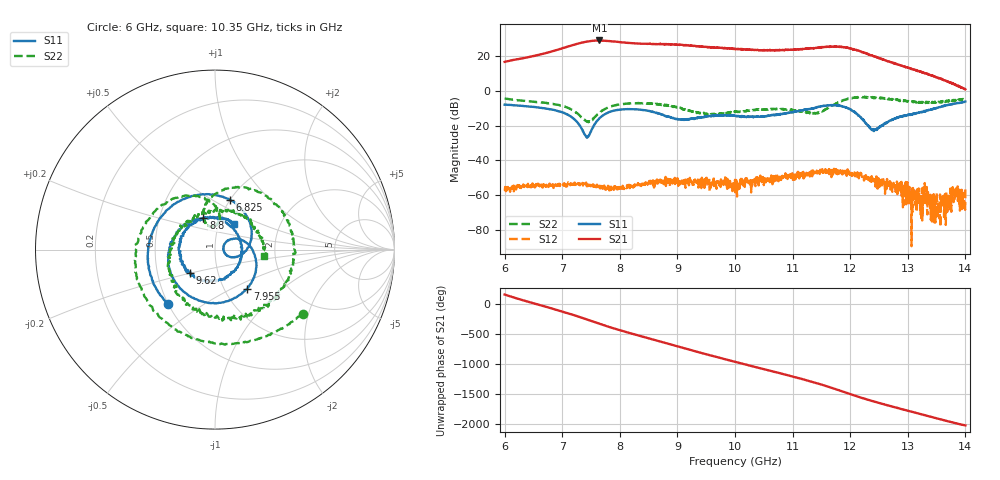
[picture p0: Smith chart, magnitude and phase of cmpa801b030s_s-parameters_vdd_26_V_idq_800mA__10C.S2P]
!Keysight Technologies,E5071C,MY46110325,B.14.03
!Date: Fri Aug 07 13:49:55 2020
!Data & Calibration Information:
!Freq	S11:SOLT2(ON)	S21:SOLT2(ON)	S12:SOLT2(ON)	S22:SOLT2(ON)
!PortZ  Port1:50+j0  Port2:50+j0
!Above PortZ is port z conversion or system Z0 setting when saving the data.
!When reading, reference impedance value at option line is always used.
# Hz S dB R 50
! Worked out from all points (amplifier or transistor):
!   1601 points, 6 GHz to 14 GHz, reference 50 ohm
!   highest |S21| = 29.0 dB at 7.645 GHz (marker M1)
!   |S21| within 3 dB of that: 7.15 GHz to 9.222 GHz (2.072 GHz wide, 25.3 % of centre)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
!   unconditionally stable (mu >= 1): start of sweep to end of sweep
!   at 7.33 GHz: K = 9.77, MAG = 27.8 dB, |S12| = -53.7 dB
!   at 10 GHz: K = 10.16, MAG = 24.5 dB, |S12| = -51.1 dB
!   at 14 GHz: K = 123.78, MAG = 4.0 dB, |S12| = -55.0 dB
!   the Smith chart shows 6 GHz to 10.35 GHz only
!   S11 on the Smith chart (normalised r, x): 6 GHz: 0.50, -0.36; 6.825 GHz: 1.00, +0.60; 7.955 GHz: 1.27, -0.61; 8.8 GHz: 0.83, +0.30; 9.62 GHz: 0.74, -0.20; 10.35 GHz: 1.19, +0.35
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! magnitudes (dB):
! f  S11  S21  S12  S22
! 6 GHz  -7.9  16.6  -57.3  -4.3
! 6.825 GHz  -10.8  22.7  -54.0  -7.5
! 7.335 GHz  -21.6  27.7  -54.0  -15.1
! 7.445 GHz  -26.4  28.3  -54.7  -17.4
! 7.645 GHz  -15.8  29.0  -55.1  -12.7
! 7.955 GHz  -10.9  28.1  -56.2  -8.0
! 8.67 GHz  -13.0  26.9  -52.8  -7.7
! 8.8 GHz  -14.5  26.9  -54.7  -8.5
! 9.62 GHz  -14.5  25.0  -52.4  -13.3
! 10 GHz  -14.4  24.1  -51.1  -12.1
! 10.35 GHz  -14.9  23.5  -52.9  -11.1
! 11.34 GHz  -10.2  24.5  -46.7  -12.9
! 11.94 GHz  -9.8  24.8  -44.9  -4.8
! 12.4 GHz  -22.3  19.8  -50.5  -3.8
! 12.67 GHz  -17.6  17.0  -54.8  -4.5
! 12.96 GHz  -14.1  13.8  -54.9  -5.8
! 13.04 GHz  -13.9  12.9  -59.1  -6.1
! 13.33 GHz  -11.4  9.8  -55.3  -6.8
! 13.52 GHz  -9.7  7.6  -63.7  -6.4
! 13.8 GHz  -7.4  3.9  -61.9  -5.5
! 13.96 GHz  -6.5  1.7  -61.7  -4.7
! 14 GHz  -6.1  0.9  -55.0  -4.5
